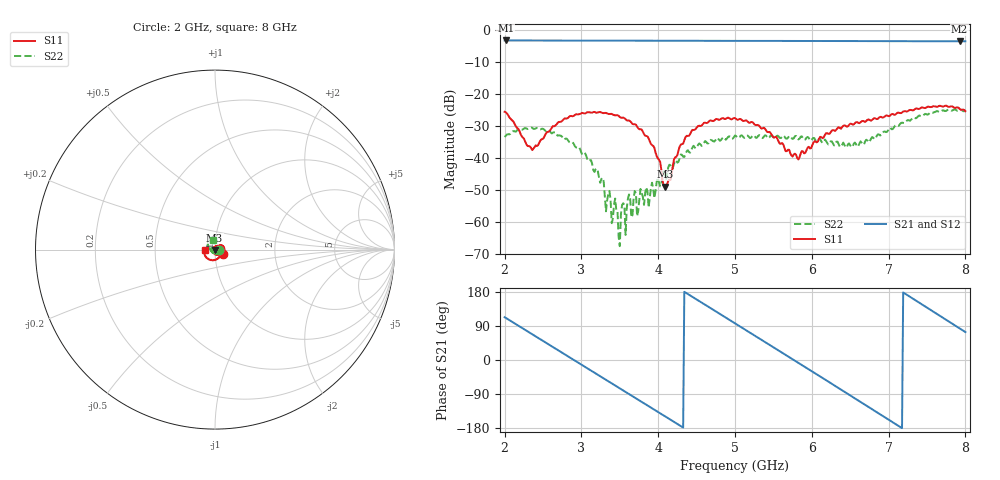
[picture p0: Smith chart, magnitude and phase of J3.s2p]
!Agilent Technologies,E8364B,MY43040699,A.07.50.67
!Agilent E8364B: A.07.50.67
!Date: Friday, June 06, 2025 05:52:12
!Correction: S11(Full 2 Port(1,2))
!S21(Full 2 Port(1,2))
!S12(Full 2 Port(1,2))
!S22(Full 2 Port(1,2))
!S2P File: Measurements: S11, S21, S12, S22:
# Hz S  dB  R 50
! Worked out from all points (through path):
!   401 points, 2 GHz to 8 GHz, reference 50 ohm
!   highest |S21| = -3.20 dB at 2.015 GHz (marker M1); lowest = -3.5 dB at 7.925 GHz (marker M2)
!   group delay of S21, straight-line fit = 351 ps
!   lowest |S11| = -49.0 dB at 4.085 GHz (marker M3), VSWR 1.01, Z = 49.8 - j0.26 ohm
!   |S11| at or under -10 dB: start of sweep to end of sweep
!   |S22| runs from -67.6 to -24.8 dB; largest |S21 - S12| = 0.0027
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2e9  -25.53 -30.3  -3.21 113.0  -3.20 113.0  -33.43 -3.3
2.015e9  -25.71 -30.6  -3.20 111.1  -3.21 111.1  -33.04 -4.2
2.36e9  -37.49 5.0  -3.22 67.9  -3.20 67.9  -30.56 -46.7
2.705e9  -28.71 41.0  -3.24 24.8  -3.23 24.8  -32.89 -84.3
3.005e9  -25.86 18.4  -3.26 -12.7  -3.25 -12.7  -38.65 -122.9
3.26e9  -25.73 -6.7  -3.26 -44.6  -3.25 -44.6  -46.55 -151.1
3.485e9  -26.79 -30.1  -3.27 -72.8  -3.26 -72.7  -64.70 25.1
3.62e9  -28.23 -43.3  -3.27 -89.7  -3.26 -89.6  -51.37 41.3
3.785e9  -31.08 -63.6  -3.28 -110.4  -3.27 -110.3  -50.92 34.1
4.01e9  -40.57 -98.8  -3.27 -138.7  -3.27 -138.6  -47.59 59.9
4.085e9  -48.95 -132.9  -3.28 -148.1  -3.28 -148.0  -45.23 65.4
4.295e9  -35.78 73.0  -3.29 -174.5  -3.30 -174.4  -38.86 61.4
4.46e9  -31.23 48.1  -3.30 164.8  -3.30 164.9  -36.16 40.8
5e9  -27.51 -23.9  -3.34 96.8  -3.33 96.9  -32.93 -30.0
5.555e9  -34.14 -117.2  -3.35 26.7  -3.35 26.8  -32.98 -119.9
5.81e9  -40.01 149.5  -3.36 -5.6  -3.36 -5.5  -33.68 -160.6
6.005e9  -36.08 89.9  -3.37 -30.3  -3.37 -30.3  -34.08 -175.3
6.5e9  -29.26 5.2  -3.37 -93.3  -3.40 -93.3  -35.98 157.7
7.01e9  -26.88 -53.6  -3.43 -158.6  -3.42 -158.6  -30.69 170.3
7.415e9  -24.41 -100.5  -3.44 149.3  -3.45 149.3  -26.85 147.7
7.925e9  -24.60 -169.4  -3.47 83.4  -3.46 83.5  -24.90 110.6
8e9  -25.32 179.9  -3.47 73.7  -3.46 73.7  -25.20 104.3
